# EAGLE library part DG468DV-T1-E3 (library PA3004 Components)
SPST Switch, TSOP-6 SMD Digikey: DG468DV-T1-E3CT-ND
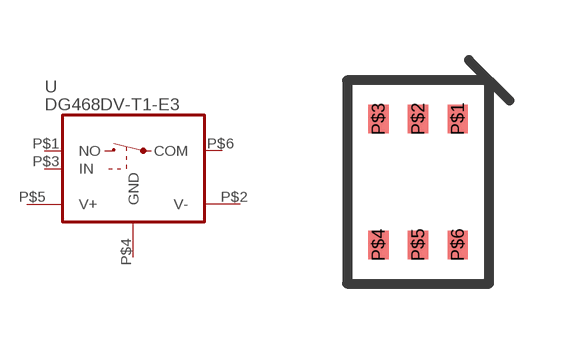
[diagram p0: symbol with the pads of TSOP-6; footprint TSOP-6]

Designator prefix -

## DG468DV-T1-E3  [TSOP-6]
P$1  NO  in
P$2  V-
P$3  IN  in
P$4  GND
P$5  V+
P$6  COM  out

## Footprint TSOP-6 (pad centres in mm)
smd 0.508 x 0.711: P$1 0.991,1.575; P$2 0,1.575; P$3 -0.991,1.575; P$4 -0.991,-1.575; P$5 0,-1.575; P$6 0.991,-1.575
